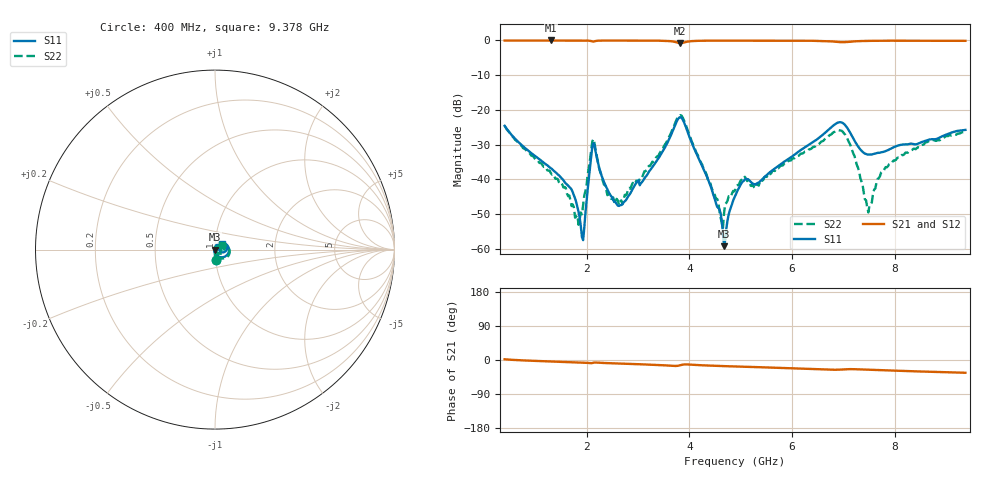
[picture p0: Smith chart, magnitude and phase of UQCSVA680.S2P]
!  Part Number  UQCSVA680  Mounting Orientation: Horizontal
!  Description: Ultra Low ESR Microwave capacitors
!  Application: Coupling, Bypass, Tuning, DC Block
!  Filters, Matching
# GHZ S DB R 50
! Freq  |S11|  S11 Ph  |S21|  S21 Ph  |S12|  S12 Ph  |S22|  S22 Ph
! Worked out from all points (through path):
!   400 points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, 400 MHz to 9.378 GHz, reference 50 ohm
!   highest |S21| = -0.01 dB at 1.3 GHz (marker M1); lowest = -0.8 dB at 3.82 GHz (marker M2)
!   group delay of S21, straight-line fit = 10.2 ps
!   lowest |S11| = -59.3 dB at 4.675 GHz (marker M3), VSWR 1.00, Z = 49.9 + j0.0216 ohm
!   |S11| at or under -10 dB: start of sweep to end of sweep
!   |S22| runs from -54.3 to -21.5 dB; largest |S21 - S12| = 0.0012
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0.4  -24.59 -86.5  -0.03 1.9  -0.03 1.9  -24.63 -86.9
1.3  -36.78 -94.1  -0.01 -3.9  -0.01 -3.9  -38.23 -90.8
1.705  -42.97 -106.3  -0.02 -5.8  -0.02 -5.8  -47.71 -74.6
1.84  -49.38 -124.0  -0.02 -6.5  -0.02 -6.5  -53.11 -29.4
1.908  -56.70 -167.7  -0.03 -6.9  -0.03 -6.9  -50.08 14.4
1.93  -57.53 148.8  -0.03 -7.0  -0.03 -7.0  -47.41 35.2
2.133  -29.61 -20.9  -0.33 -7.2  -0.33 -7.2  -28.43 -21.9
2.403  -42.93 -119.9  -0.04 -8.3  -0.03 -8.3  -44.58 -57.6
2.628  -47.68 -174.4  -0.04 -9.3  -0.04 -9.3  -47.36 -14.2
3.393  -34.04 79.5  -0.07 -13.2  -0.07 -13.2  -33.28 47.5
3.82  -22.10 -2.7  -0.78 -13.9  -0.78 -13.9  -21.52 -12.5
4.585  -48.63 -90.6  -0.06 -15.8  -0.06 -15.9  -49.11 -53.3
4.653  -55.37 -138.9  -0.07 -16.1  -0.07 -16.1  -54.28 4.8
4.675  -59.27 168.5  -0.07 -16.2  -0.07 -16.2  -49.84 30.9
4.9  -44.50 55.4  -0.06 -17.3  -0.06 -17.3  -42.80 43.7
6.408  -29.30 49.6  -0.11 -23.7  -0.10 -23.8  -30.72 56.8
6.993  -23.83 -0.4  -0.51 -24.8  -0.51 -24.8  -26.37 -16.6
7.218  -28.87 -22.0  -0.27 -24.3  -0.27 -24.3  -33.35 -56.4
7.488  -32.89 2.5  -0.14 -25.7  -0.14 -25.7  -49.55 3.2
7.668  -32.40 16.8  -0.11 -26.6  -0.10 -26.6  -39.86 52.8
7.893  -31.40 28.7  -0.08 -27.6  -0.08 -27.6  -35.64 52.4
9.378  -25.78 38.3  -0.12 -33.7  -0.11 -33.7  -26.14 34.5
